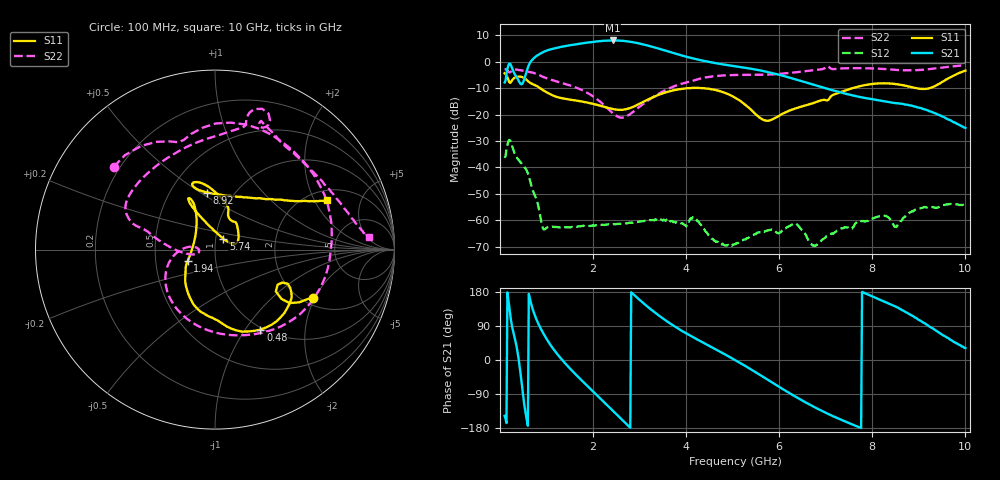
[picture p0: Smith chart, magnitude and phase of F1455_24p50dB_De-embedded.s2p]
! Integrated Device Technology
! Corporate Headquarters
! 6024 Silver Creek Valley Road
! San Jose, CA 95138  USA
! Phone:  1-408-284-8200
! Toll Free:  1-800-223-1366
! Webpage:  http://www.idt.com/
! Timing and RF Division
! 515 Groton Road, Suite 102
! Westford, MA 01886-6024
! Device:  F1455
! Description: 6-bit 0.5 dB Transmit Variable Gain Amplifier
! Frequency:  1400.0 -  2300.00 MHz
! Package:  6x6 mm Thin QFN Plastic Package: 28 pin
! State:  49
! Atten State:  24.5 dB
! Voltage:  +5.00 Volts
! Current:  217.631 mA
! Data:  The device was measured on a the F1455 evaluation board which has
!  individual transmission lines to the RF pins.  Data was collected
!  using a calibrated network analyzer.  The evaluation board was
!  de-embedded using a TRL calibration technique.
!  The reference plane is the edge of the package pin.
!  Pin  1 = CSb
!  Pin  2 = DATA
!  Pin  3 = CLK
!  Pin  4 = RSET
!  Pin  5 = GND
!  Pin  6 = RFIN  = Port 1
!  Pin  7 = GND
!  Pin  8 = NC
!  Pin  9 = NC
!  Pin 10 = NC
!  Pin 11 = NC
!  Pin 12 = NC
!  Pin 13 = NC
!  Pin 14 = /STBY
!  Pin 15 = GND
!  Pin 16 = RFOUT  = Port 2
!  Pin 17 = GND
!  Pin 18 = NC
!  Pin 19 = NC
!  Pin 20 = NC
!  Pin 21 = GND
!  Pin 22 = NC
!  Pin 23 = GND
!  Pin 24 = NC
!  Pin 25 = NC
!  Pin 26 = NC
!  Pin 27 = GND
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# GHz S dB R 50
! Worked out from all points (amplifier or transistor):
!   496 points, 100 MHz to 10 GHz, reference 50 ohm
!   highest |S21| = 8.1 dB at 2.42 GHz (marker M1)
!   |S21| within 3 dB of that: 1.171 GHz to 3.392 GHz (2.222 GHz wide, 97.4 % of centre)
!   unconditionally stable (mu >= 1): start of sweep to end of sweep
!   at 1.74 GHz: K = 256.31, MAG = 7.5 dB, |S12| = -62.2 dB
!   at 5.06 GHz: K = 1119.68, MAG = 0.2 dB, |S12| = -69.0 dB
!   at 10 GHz: K = 622.98, MAG = -16.4 dB, |S12| = -54.2 dB
!   S11 on the Smith chart (normalised r, x): 100 MHz: 2.27, -1.93; 480 MHz: 0.97, -1.18; 1.94 GHz: 0.73, -0.09; 5.74 GHz: 1.09, +0.13; 8.92 GHz: 0.75, +0.53; 10 GHz: 2.46, +2.53
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0.1  -4.31 -26.1  -7.80 -147.5  -36.36 47.4  -2.75 140.7
0.18  -6.73 -36.5  -1.33 160.4  -30.19 -6.8  -3.71 112.6
0.26  -6.96 -25.2  -2.35 88.4  -31.71 -77.1  -3.32 96.0
0.38  -5.62 -42.4  -6.42 19.6  -36.69 -118.0  -3.02 58.1
0.48  -5.80 -60.4  -8.33 -76.1  -38.82 -149.6  -3.28 31.8
0.66  -8.08 -88.0  0.04 153.2  -45.91 141.3  -3.92 -10.0
0.8  -9.21 -105.9  2.40 102.4  -52.89 111.7  -4.66 -41.1
0.96  -11.11 -123.5  3.95 64.2  -63.44 128.2  -5.93 -70.5
1.34  -13.80 -143.6  5.76 -0.2  -62.56 109.6  -8.03 -120.9
1.76  -15.00 -153.7  7.00 -54.4  -62.12 79.9  -10.66 -157.6
1.94  -15.68 -157.7  7.44 -75.9  -62.14 71.4  -12.38 -170.0
2.18  -16.75 -166.0  7.91 -104.4  -61.74 61.3  -15.48 176.9
2.42  -17.85 179.6  8.10 -133.4  -61.54 53.6  -19.37 173.3
2.82  -17.32 142.9  7.55 178.8  -60.82 43.7  -19.50 -167.3
3.4  -12.54 117.0  5.06 118.7  -59.70 24.3  -12.21 177.2
4.08  -9.92 116.3  1.58 64.9  -59.63 11.9  -7.45 163.6
5.06  -13.61 114.5  -1.68 -0.6  -69.04 23.1  -4.96 148.6
5.74  -22.32 52.0  -3.78 -51.0  -63.92 23.1  -4.84 120.4
6.7  -15.80 37.1  -8.44 -120.7  -69.13 -141.8  -3.25 78.7
8.36  -8.18 108.5  -15.28 148.5  -59.12 71.8  -2.84 62.8
8.92  -9.87 97.8  -16.96 111.9  -55.97 91.2  -3.16 40.3
10  -3.33 23.9  -25.04 31.4  -54.17 20.2  -1.28 4.7
